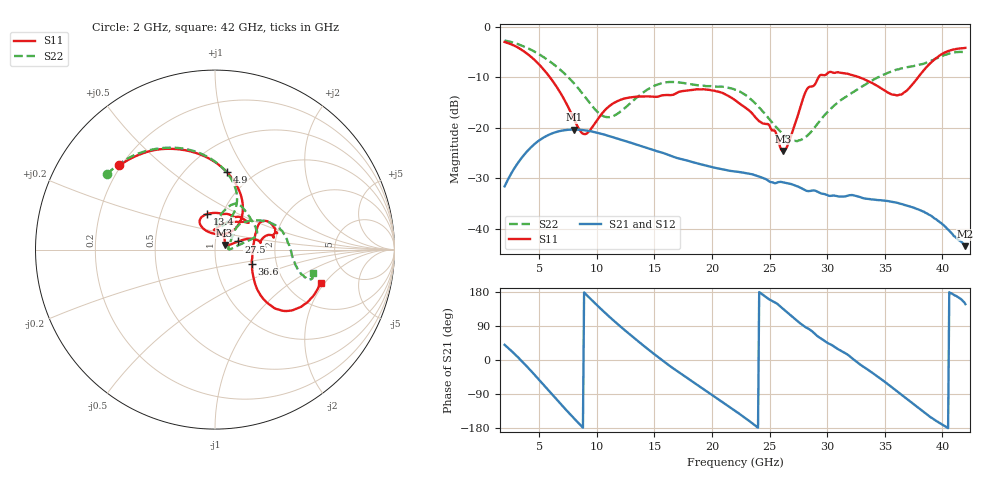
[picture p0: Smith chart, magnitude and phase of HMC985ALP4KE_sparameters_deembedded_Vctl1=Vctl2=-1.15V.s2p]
!s2p File: Measurements: S11, S21, S12, S22
# GHz S dB R 50.0
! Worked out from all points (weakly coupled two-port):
!   401 points, 2 GHz to 42 GHz, reference 50 ohm
!   highest |S21| = -20.34 dB at 8 GHz (marker M1); lowest = -43.5 dB at 42 GHz (marker M2)
!   lowest |S11| = -24.6 dB at 26.2 GHz (marker M3), VSWR 1.12, Z = 55.5 + j2.84 ohm
!   |S11| at or under -10 dB: 5.939 GHz to 29.25 GHz (23.31 GHz wide, 132 % of centre); 32.78 GHz to 37.89 GHz (5.109 GHz wide, 14.5 % of centre)
!   |S22| runs from -22.6 to -2.7 dB; largest |S21 - S12| = 0.00013
!   S11 on the Smith chart (normalised r, x): 2 GHz: 0.19, +0.37; 4.9 GHz: 0.77, +0.82; 13.4 GHz: 0.85, +0.35; 27.5 GHz: 1.29, +0.12; 36.6 GHz: 1.49, -0.25; 42 GHz: 3.03, -1.86
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2  -2.98 138.6  -31.61 39.9  -31.62 39.9  -2.68 145.2
3.4  -4.43 111.2  -26.20 -0.1  -26.20 -0.1  -3.62 122.3
4.9  -7.22 81.0  -22.67 -49.1  -22.67 -49.1  -5.29 98.9
6.2  -10.82 57.4  -21.04 -93.4  -21.05 -93.5  -7.31 80.8
8  -18.17 50.6  -20.34 -153.3  -20.35 -153.3  -11.12 64.4
8.7  -21.00 72.0  -20.43 -175.4  -20.43 -175.4  -13.04 62.8
10.9  -16.08 120.5  -21.52 119.5  -21.52 119.5  -17.89 80.9
13.4  -13.84 102.3  -23.29 54.1  -23.30 54.1  -14.14 80.7
15.4  -13.75 75.5  -24.75 6.2  -24.75 6.1  -11.31 68.5
18.9  -12.39 39.8  -27.16 -69.4  -27.17 -69.3  -11.60 41.7
22  -14.51 55.2  -28.66 -133.9  -28.67 -133.9  -12.43 18.1
24.9  -19.31 88.8  -30.50 161.0  -30.50 161.0  -18.08 9.5
26.2  -24.62 25.7  -30.81 134.2  -30.81 134.2  -21.36 1.6
27.5  -17.21 19.1  -31.68 100.8  -31.70 100.6  -22.55 6.4
28.2  -12.54 13.6  -32.49 85.2  -32.47 85.3  -21.71 17.7
28.7  -11.79 8.8  -32.44 75.5  -32.44 75.5  -20.53 25.9
31  -9.01 19.8  -33.61 27.7  -33.63 27.7  -14.84 46.1
33.3  -10.46 31.1  -34.03 -20.8  -34.01 -20.9  -11.45 37.2
35.4  -13.14 10.3  -34.60 -67.2  -34.59 -67.0  -9.01 23.5
36.6  -13.13 -21.0  -35.19 -95.1  -35.22 -95.0  -8.17 14.3
39.6  -5.95 -42.4  -38.43 -162.9  -38.41 -163.3  -6.15 -15.2
42  -4.15 -17.7  -43.47 147.5  -43.46 147.7  -5.03 -13.2
